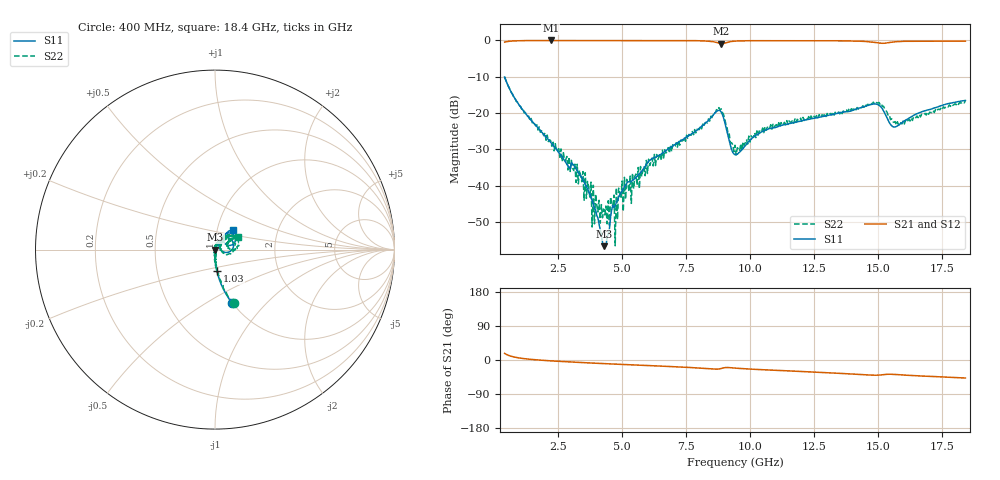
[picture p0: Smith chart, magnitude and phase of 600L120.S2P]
!  American Technical Ceramics  Date:  10/27/06
!  One Norden Lane
!  Huntington Station,  NY.  11746-2102
!  Tel:  (631) 622-4700  Fax:  (631) 622-4748
!  Part Number  600L120		Mounting Orientation: Vertical
!  Description: Ultra Low ESR Microwave capacitors
!  Application: Coupling, Bypass, Tuning, DC Block
!  Filters, Matching
# GHZ S DB R 50
! Freq  |S11|  S11 Ph  |S21|  S21 Ph  |S12|  S12 Ph  |S22|  S22 Ph
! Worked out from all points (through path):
!   401 points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, 400 MHz to 18.4 GHz, reference 50 ohm
!   highest |S21| = -0.02 dB at 2.2 GHz (marker M1); lowest = -0.9 dB at 8.86 GHz (marker M2)
!   group delay of S21, straight-line fit = 7.95 ps
!   lowest |S11| = -56.7 dB at 4.27 GHz (marker M3), VSWR 1.00, Z = 50.1 - j0.0704 ohm
!   |S11| at or under -10 dB: start of sweep to end of sweep
!   |S22| runs from -56.6 to -10.0 dB; largest |S21 - S12| = 0.0029
!   S11 on the Smith chart (normalised r, x): 400 MHz: 0.99, -0.66; 1.03 GHz: 0.99, -0.24; 18.4 GHz: 1.19, +0.27
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0.4  -10.09 -72.3  -0.49 17.4  -0.48 17.4  -10.00 -70.9
1.03  -18.42 -85.2  -0.08 4.8  -0.07 4.8  -18.23 -82.5
2.2  -28.10 -90.9  -0.02 -2.2  -0.02 -2.3  -27.64 -83.2
3.415  -37.79 -94.7  -0.03 -6.8  -0.02 -6.8  -38.95 -113.6
3.685  -41.72 -92.2  -0.03 -7.6  -0.02 -7.7  -40.41 -64.3
3.91  -46.19 -83.8  -0.03 -8.3  -0.02 -8.4  -50.53 -44.8
4.27  -56.68 -28.6  -0.03 -9.5  -0.02 -9.5  -46.45 -175.4
4.405  -54.24 27.3  -0.03 -9.9  -0.02 -9.9  -50.54 -72.4
4.585  -46.55 60.2  -0.03 -10.4  -0.02 -10.5  -45.59 126.5
4.72  -45.46 54.7  -0.03 -10.9  -0.03 -10.9  -56.58 7.8
4.81  -44.04 59.1  -0.03 -11.2  -0.03 -11.2  -49.35 129.2
4.855  -43.12 60.8  -0.03 -11.3  -0.03 -11.3  -40.69 52.7
5.08  -40.28 63.0  -0.04 -12.0  -0.03 -12.0  -37.72 71.2
6.43  -31.65 64.4  -0.04 -15.9  -0.04 -16.0  -32.11 63.9
8.86  -19.74 7.5  -0.89 -22.5  -0.90 -22.6  -18.84 0.3
9.4  -31.47 18.2  -0.20 -21.3  -0.21 -21.5  -28.89 6.0
10.525  -24.93 58.9  -0.09 -25.8  -0.09 -25.9  -25.40 50.2
12.415  -21.54 57.8  -0.08 -31.7  -0.08 -31.8  -21.54 54.2
14.845  -17.51 36.7  -0.53 -40.2  -0.53 -40.2  -17.42 26.1
15.43  -22.66 19.7  -0.59 -37.6  -0.60 -37.6  -20.59 0.8
15.925  -22.67 51.6  -0.28 -39.3  -0.28 -39.3  -23.00 19.2
18.4  -16.53 47.4  -0.22 -47.5  -0.24 -47.5  -16.63 28.8
